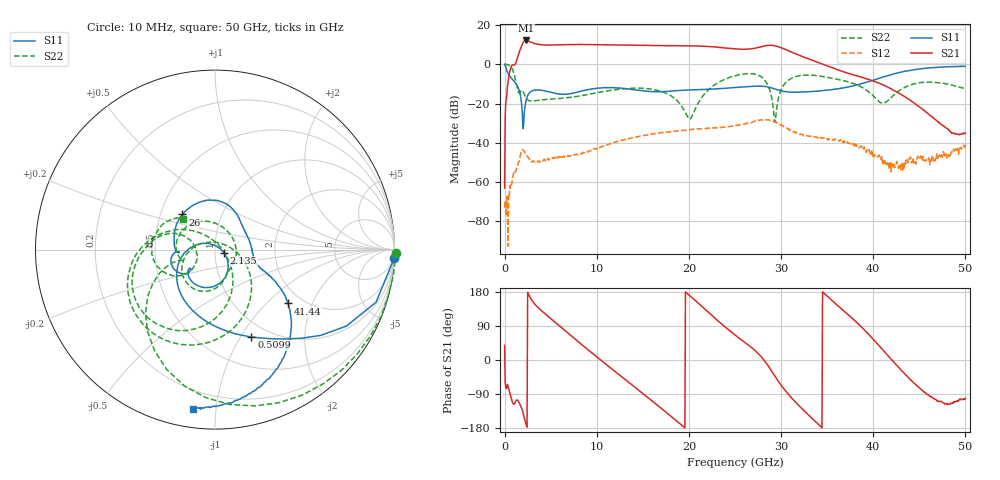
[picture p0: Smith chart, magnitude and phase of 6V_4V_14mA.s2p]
! MARKI MICROWAVE INC.
! Date:  1/07/2020
! Model Number:  APM-6849CH
! Description:  2-port Small Signal S-parameter data for APM-6849CH
! Frequency Range:  10 MHz to 50 GHz
! Port Configuration:  PORT 1: Input
!  PORT 2: Output
! Bias Condition: Vc = +6V, Vb = +4V
! APM-6849CH s2p files are only valid for small signal conditions (below -5 dBm input power)
!S2P File: Measurements: Mag<S11> Ang<S11>, Mag<S21> Ang<S21>, Mag<S12> Ang<S12>, Mag<S22> Ang<S22>!row 1
# Hz S  dB  R 50
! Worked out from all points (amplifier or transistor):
!   801 points, 10 MHz to 50 GHz, reference 50 ohm
!   highest |S21| = 12.2 dB at 2.322 GHz (marker M1)
!   |S21| within 3 dB of that: 1.84 GHz to 21.89 GHz (20.05 GHz wide, 169 % of centre)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
!   unconditionally stable (mu >= 1): 128.9 MHz to end of sweep
!   at 8.321 GHz: K = 27.71, MAG = 10.4 dB, |S12| = -45.6 dB
!   at 25 GHz: K = 5.16, MAG = 9.5 dB, |S12| = -31.3 dB
!   at 50 GHz: K = 593.54, MAG = -27.8 dB, |S12| = -41.0 dB
!   S11 on the Smith chart (normalised r, x): 10 MHz: 1, -41; 509.9 MHz: 0.83, -1.12; 2.135 GHz: 1.10, -0.04; 26 GHz: 0.65, +0.27; 41.44 GHz: 1.69, -1.36; 50 GHz: 0.10, -0.87
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1e7  -0.01 -2.8  -63.07 39.0  -72.99 -98.6  0.06 -1.1
5.099e8  -5.56 -67.4  -5.03 -80.6  -67.82 48.7  -0.49 -59.0
1.5097e9  -12.19 -150.1  5.17 -109.0  -50.05 -72.2  -14.24 -162.2
2.134575e9  -25.51 -19.2  11.85 -151.3  -44.34 -147.5  -15.11 115.7
2.322038e9  -18.63 -50.8  12.17 -168.1  -45.32 -164.9  -16.96 83.9
3.071888e9  -13.40 -99.1  10.89 153.8  -49.18 177.7  -18.69 11.3
4.634075e9  -13.79 -137.0  9.84 117.0  -48.82 169.4  -17.80 -33.8
8.383325e9  -13.58 -140.5  10.11 40.4  -45.58 133.2  -15.94 -67.2
1.175765e10  -11.88 -163.8  9.90 -25.8  -40.22 102.8  -13.08 -92.3
1.431964e10  -13.10 -176.2  9.73 -75.3  -36.91 67.8  -12.10 -118.7
1.669416e10  -13.98 -175.8  9.57 -121.4  -35.12 33.4  -13.36 -149.4
2.031844e10  -13.00 177.0  9.42 165.1  -33.07 -21.1  -26.71 50.7
2.263048e10  -12.56 165.9  8.92 114.7  -32.32 -61.3  -11.00 -44.0
2.5005e10  -11.81 146.0  7.86 65.8  -31.30 -103.4  -5.82 -92.3
2.60048e10  -11.47 132.9  7.66 47.4  -30.42 -126.6  -4.91 -113.8
2.844181e10  -11.41 82.5  9.61 -10.0  -28.27 156.1  -9.51 166.5
2.987902e10  -13.32 50.7  8.71 -62.3  -30.62 100.4  -14.50 -58.6
3.337832e10  -13.82 2.1  2.03 -154.5  -36.52 28.0  -5.55 -144.3
3.662768e10  -12.07 -19.7  -3.55 133.4  -39.11 -38.9  -8.18 179.3
4.143921e10  -5.92 -36.3  -11.29 16.0  -50.96 165.2  -19.04 -154.5
4.168916e10  -5.60 -38.1  -11.84 9.2  -51.10 151.4  -18.07 -146.9
5e10  -0.96 -98.0  -35.07 -101.1  -41.01 -58.2  -12.20 136.8
